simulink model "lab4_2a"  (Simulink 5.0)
settings: Solver=FixedStepDiscrete  StartTime=0.0  StopTime=2*1e-3  FixedStep=T  RelTol=1e-3
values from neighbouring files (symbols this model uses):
  T = 1/Fsamp    (= 0.0001)    [lab4_4.m]

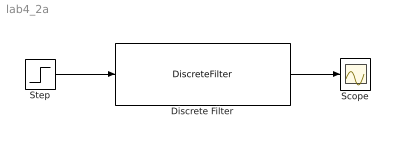
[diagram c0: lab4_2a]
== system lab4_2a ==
  Discrete Filter : DiscreteFilter  Numerator="[2  1]"  Denominator="[1  -1.8*cos(pi/16)  0.81]"  SampleTime=T
  Scope : Scope
  Step : Step  Time=0  SampleTime=0
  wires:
  Discrete Filter/1 -> Scope/1
  Step/1 -> Discrete Filter/1
